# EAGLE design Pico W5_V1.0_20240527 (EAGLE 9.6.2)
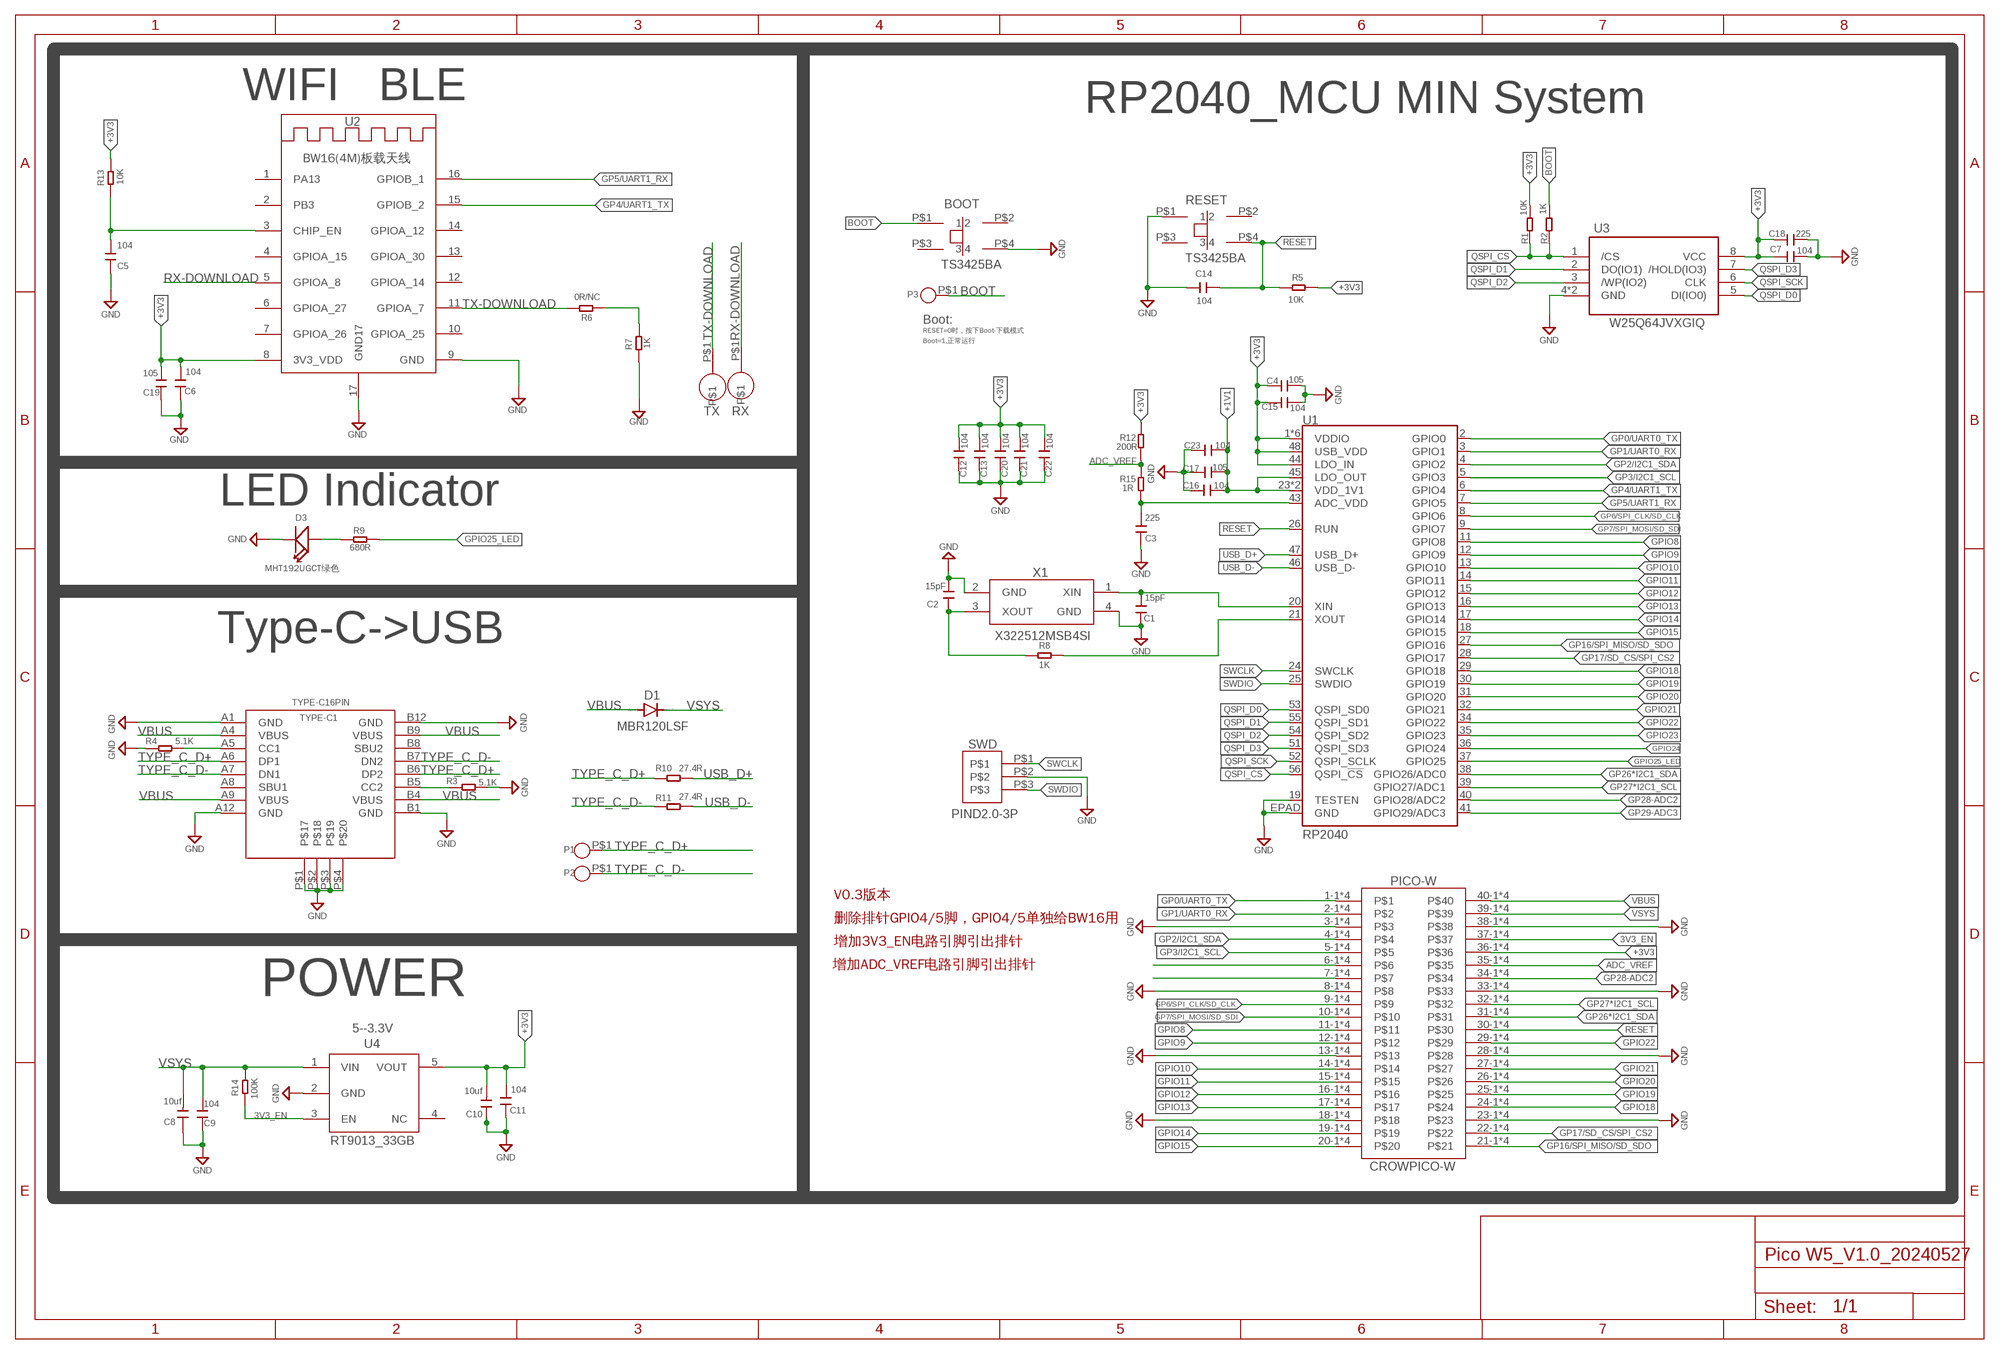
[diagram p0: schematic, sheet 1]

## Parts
BOOT  TS3425BA  KEY  [SMD_KEY4.2*3.*.2.5]
C1  15pF  C0201  [0201_W]
C2  15pF  C0201  [0201_W]
C3  225  C0201  [0201_W]
C4  105  C0201  [0201_W]
C5  104  C0201  [0201_W]
C6  104  C0201  [0201_W]
C7  104  C0201  [0201_W]
C8  10uf  C0402  [0402]
C9  104  C0402  [0201_W]
C10  10uf  C0402  [0402]
C11  104  C0402  [0201_W]
C12  104  C0201  [0201_W]
C13  104  C0201  [0201_W]
C14  104  C0402  [0201_W]
C15  104  C0201  [0201_W]
C16  104  C0201  [0201_W]
C17  105  C0201  [0201_W]
C18  225  C0201  [0201_W]
C19  105  C0201  [0201_W]
C20  104  C0201  [0201_W]
C21  104  C0201  [0201_W]
C22  104  C0201  [0201_W]
C23  104  C0201  [0201_W]
D1  MBR120LSF  DIODE-SOD123  [SOD123]
D3  MHT192UGCT绿色  DISCRETE_007-LED0603  [DISCRETE_D0603]
P1  TP  CROWPICO_W_PAD-1P  [CROWPICO_W_PAD-1P]
P2  TP  CROWPICO_W_PAD-1P  [CROWPICO_W_PAD-1P]
P3  TP  CROWPICO_W_PAD-1P  [CROWPICO_W_PAD-1P]
PICO-W  CROWPICO-W  CROWPICO-WCROWPICO-W1  [CROWPICO-W]
R1  10K  R0201  [0201_W]
R2  1K  R0201  [0201_W]
R3  5.1K  R0201  [0201_W]
R4  5.1K  R0201  [0201_W]
R5  10K  R0201  [0201_W]
R6  0R/NC  R0201  [0201_W]
R7  1K  R0201  [0201_W]
R8  1K  R0201  [0201_W]
R9  680R  R0201  [0201_W]
R10  27.4R  R0201  [0201_W]
R11  27.4R  R0201  [0201_W]
R12  200R  R0201  [0201_W]
R13  10K  R0201  [0201_W]
R14  100K  R0201  [0201_W]
R15  1R  R0201  [0201_W]
RESET  TS3425BA  KEY  [SMD_KEY4.2*3.*.2.5]
RX  TP  [TP2]
SWD  PIND2.0-3P  PIND2.0  [HDR2.0-3P]
TX  TP  [TP2]
TYPE-C1  TYPE-C16PIN  TYPE-C-16PIN  [TYPE-C16PIN2MD(073)]
U1  RP2040  RP2040_RP2040  [RP2040_QFN-56]
U2  BW16(4M)板载天线  BW16  [BW16]
U3  W25Q64JVXGIQ  W25QXX  [W25QXX-XSON-8-EP(4X4)]
U4  RT9013_33GB  RT9013  [SOT23-5_W]
X1  X322512MSB4SI  A_XBJ_XTAL  [A_XBJ_SMD3225]

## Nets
3V3_EN: PICO-W.37-1 PICO-W.37-2 PICO-W.37-3 PICO-W.37-4 R14.1 U4.3(EN)
+1V1: C16.1 C17.1 C23.1 U1.23(VDD_1V1) U1.45(LDO_OUT) U1.50(VDD_1V1)
+3V3: C4.2 C6.2 C7.1 C10.2 C11.2 C12.1 C13.1 C15.2 C18.1 C19.2 C20.1 C21.1 C22.1 PICO-W.36-1 PICO-W.36-2 PICO-W.36-3 PICO-W.36-4 R1.2 R5.2 R12.2 R13.2 U1.1(VDDIO) U1.10(VDDIO) U1.22(VDDIO) U1.33(VDDIO) U1.42(VDDIO) U1.44(LDO_IN) U1.48(USB_VDD) U1.49(VDDIO) U2.8(3V3_VDD) U3.8(VCC) U4.5(VOUT)
ADC_VREF: PICO-W.35-1 PICO-W.35-2 PICO-W.35-3 PICO-W.35-4 R12.1 R15.2
BOOT: BOOT.P$1 P3.P$1 R2.2
GND: BOOT.P$4 C1.2 C2.1 C3.2 C4.1 C5.1 C6.1 C7.2 C8.1 C9.1 C10.1 C11.1 C12.2 C13.2 C14.1 C15.1 C16.2 C17.2 C18.2 C19.1 C20.2 C21.2 C22.2 C23.2 D3.- PICO-W.3-1 PICO-W.3-2 PICO-W.3-3 PICO-W.3-4 PICO-W.8-1 PICO-W.8-2 PICO-W.8-3 PICO-W.8-4 PICO-W.13-1 PICO-W.13-2 PICO-W.13-3 PICO-W.13-4 PICO-W.18-1 PICO-W.18-2 PICO-W.18-3 PICO-W.18-4 PICO-W.23-1 PICO-W.23-2 PICO-W.23-3 PICO-W.23-4 PICO-W.28-1 PICO-W.28-2 PICO-W.28-3 PICO-W.28-4 PICO-W.33-1 PICO-W.33-2 PICO-W.33-3 PICO-W.33-4 PICO-W.38-1 PICO-W.38-2 PICO-W.38-3 PICO-W.38-4 R3.2 R4.1 R7.1 RESET.P$1 SWD.P$2 TYPE-C1.A1(GND) TYPE-C1.A12(GND) TYPE-C1.B1(GND) TYPE-C1.B12(GND) TYPE-C1.P$1 TYPE-C1.P$2 TYPE-C1.P$3 TYPE-C1.P$4 U1.19(TESTEN) U1.EPAD(GND) U2.9(GND) U2.17(GND17) U3.4(GND) U3.EP(GND) U4.2(GND) X1.2(GND) X1.4(GND)
GP0/UART0_TX: PICO-W.1-1 PICO-W.1-2 PICO-W.1-3 PICO-W.1-4 U1.2(GPIO0)
GP1/UART0_RX: PICO-W.2-1 PICO-W.2-2 PICO-W.2-3 PICO-W.2-4 U1.3(GPIO1)
GP2/I2C1_SDA: PICO-W.4-1 PICO-W.4-2 PICO-W.4-3 PICO-W.4-4 U1.4(GPIO2)
GP3/I2C1_SCL: PICO-W.5-1 PICO-W.5-2 PICO-W.5-3 PICO-W.5-4 U1.5(GPIO3)
GP4/UART1_TX: U1.6(GPIO4) U2.15(GPIOB_2)
GP5/UART1_RX: U1.7(GPIO5) U2.16(GPIOB_1)
GP6/SPI_CLK/SD_CLK: PICO-W.9-1 PICO-W.9-2 PICO-W.9-3 PICO-W.9-4 U1.8(GPIO6)
GP7/SPI_MOSI/SD_SDI: PICO-W.10-1 PICO-W.10-2 PICO-W.10-3 PICO-W.10-4 U1.9(GPIO7)
GP16/SPI_MISO/SD_SDO: PICO-W.21-1 PICO-W.21-2 PICO-W.21-3 PICO-W.21-4 U1.27(GPIO16)
GP17/SD_CS/SPI_CS2: PICO-W.22-1 PICO-W.22-2 PICO-W.22-3 PICO-W.22-4 U1.28(GPIO17)
GP26*I2C1_SDA: PICO-W.31-1 PICO-W.31-2 PICO-W.31-3 PICO-W.31-4 U1.38(GPIO26/ADC0)
GP27*I2C1_SCL: PICO-W.32-1 PICO-W.32-2 PICO-W.32-3 PICO-W.32-4 U1.39(GPIO27/ADC1)
GP28-ADC2: PICO-W.34-1 PICO-W.34-2 PICO-W.34-3 PICO-W.34-4 U1.40(GPIO28/ADC2)
GP29-ADC3: U1.41(GPIO29/ADC3)
GPIO8: PICO-W.11-1 PICO-W.11-2 PICO-W.11-3 PICO-W.11-4 U1.11(GPIO8)
GPIO9: PICO-W.12-1 PICO-W.12-2 PICO-W.12-3 PICO-W.12-4 U1.12(GPIO9)
GPIO10: PICO-W.14-1 PICO-W.14-2 PICO-W.14-3 PICO-W.14-4 U1.13(GPIO10)
GPIO11: PICO-W.15-1 PICO-W.15-2 PICO-W.15-3 PICO-W.15-4 U1.14(GPIO11)
GPIO12: PICO-W.16-1 PICO-W.16-2 PICO-W.16-3 PICO-W.16-4 U1.15(GPIO12)
GPIO13: PICO-W.17-1 PICO-W.17-2 PICO-W.17-3 PICO-W.17-4 U1.16(GPIO13)
GPIO14: PICO-W.19-1 PICO-W.19-2 PICO-W.19-3 PICO-W.19-4 U1.17(GPIO14)
GPIO15: PICO-W.20-1 PICO-W.20-2 PICO-W.20-3 PICO-W.20-4 U1.18(GPIO15)
GPIO18: PICO-W.24-1 PICO-W.24-2 PICO-W.24-3 PICO-W.24-4 U1.29(GPIO18)
GPIO19: PICO-W.25-1 PICO-W.25-2 PICO-W.25-3 PICO-W.25-4 U1.30(GPIO19)
GPIO20: PICO-W.26-1 PICO-W.26-2 PICO-W.26-3 PICO-W.26-4 U1.31(GPIO20)
GPIO21: PICO-W.27-1 PICO-W.27-2 PICO-W.27-3 PICO-W.27-4 U1.32(GPIO21)
GPIO22: PICO-W.29-1 PICO-W.29-2 PICO-W.29-3 PICO-W.29-4 U1.34(GPIO22)
GPIO23: U1.35(GPIO23)
GPIO24: U1.36(GPIO24)
GPIO25_LED: R9.2 U1.37(GPIO25)
N$1: C2.2 R8.1 X1.3(XOUT)
N$2: R8.2 U1.21(XOUT)
N$3: C1.1 U1.20(XIN) X1.1(XIN)
N$4: C3.1 R15.1 U1.43(ADC_VDD)
N$5: R3.1 TYPE-C1.B5(CC2)
N$7: R6.1 R7.2
N$8: PICO-W.6-1 PICO-W.6-2 PICO-W.6-3 PICO-W.6-4
N$9: PICO-W.7-1 PICO-W.7-2 PICO-W.7-3 PICO-W.7-4
N$14: R4.2 TYPE-C1.A5(CC1)
N$16: C5.2 R13.1 U2.3(CHIP_EN)
N$35: D3.+ R9.1
QSPI_CS: R1.1 R2.1 U1.56(QSPI_!CS!) U3.1(/CS)
QSPI_D0: U1.53(QSPI_SD0) U3.5(DI(IO0))
QSPI_D1: U1.55(QSPI_SD1) U3.2(DO(IO1))
QSPI_D2: U1.54(QSPI_SD2) U3.3(/WP(IO2))
QSPI_D3: U1.51(QSPI_SD3) U3.7(/HOLD(IO3))
QSPI_SCK: U1.52(QSPI_SCLK) U3.6(CLK)
RESET: C14.2 PICO-W.30-1 PICO-W.30-2 PICO-W.30-3 PICO-W.30-4 R5.1 RESET.P$4 U1.26(RUN)
RX-DOWNLOAD: RX.P$1 U2.5(GPIOA_8)
SWCLK: SWD.P$1 U1.24(SWCLK)
SWDIO: SWD.P$3 U1.25(SWDIO)
TX-DOWNLOAD: R6.2 TX.P$1 U2.11(GPIOA_7)
TYPE_C_D+: P1.P$1 R10.1 TYPE-C1.A6(DP1) TYPE-C1.B6(DP2)
TYPE_C_D-: P2.P$1 R11.1 TYPE-C1.A7(DN1) TYPE-C1.B7(DN2)
USB_D+ [USB]: R10.2 U1.47(USB_D+)
USB_D- [USB]: R11.2 U1.46(USB_D-)
VBUS [PWR]: D1.A PICO-W.40-1 PICO-W.40-2 PICO-W.40-3 PICO-W.40-4 TYPE-C1.A4(VBUS) TYPE-C1.A9(VBUS) TYPE-C1.B4(VBUS) TYPE-C1.B9(VBUS)
VSYS: C8.2 C9.2 D1.C PICO-W.39-1 PICO-W.39-2 PICO-W.39-3 PICO-W.39-4 R14.2 U4.1(VIN)
Unconnected: BOOT.P$2 BOOT.P$3 RESET.P$2 RESET.P$3 TYPE-C1.A8(SBU1) TYPE-C1.B8(SBU2) U2.1(PA13) U2.2(PB3) U2.4(GPIOA_15) U2.6(GPIOA_27) U2.7(GPIOA_26) U2.10(GPIOA_25) U2.12(GPIOA_14) U2.13(GPIOA_30) U2.14(GPIOA_12) U4.4(NC)

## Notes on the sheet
- WIFI   BLE | RP2040_MCU MIN System
- Boot:
- RESET=0时，按下Boot-下载模式
- Boot=1,正常运行
- LED Indicator
- Type-C->USB
- V0.3版本
- 删除排针GPIO4/5脚，GPIO4/5单独给BW16用
- 增加3V3_EN电路引脚引出排针
- 增加ADC_VREF电路引脚引出排针
- POWER
- 5--3.3V

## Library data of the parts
BOOT RESET = CKP:KEY
C1-C7 C12 C13 C15-C23 = WGH:C0201
C8 C10 = A_xbj:C0402
C9 C11 C14 = WGH:C0402
D1 = diode:DIODE-: DIODE
D3 = Crowtail_SIM1606:DISCRETE_007-LED*
P1-P3 = ESP32- 3.5 TFT Display(RGB)-V2.0:CROWPICO_W_PAD-1P
PICO-W = CKP:CROWPICO-W
R1-R15 = WGH:R0201
RX TX = CKP:TP
SWD = CKP:PIND2.0
TYPE-C1 = CKP:TYPE-C-16PIN
U1 = Lora_RA-08H_Dev:RP2040_RP2040: Raspberry Pi RP2040 MCU 56-pin 32-bit Microcontroller with 264kB of SRAM and external flash support up to 16MB Getting Started with the RP2040 Dual-core ARM Cortex M0+ processor, flexible clock running up to 133 MHz 264kB of SRAM, and QSPI control of common flash memory USB 1.1 Host and Device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; PROD_ID: IC-15502
U2 = CKP:BW16
U3 = CKP:W25QXX
U4 = WGH:RT9013
X1 = CrowBot_V1.4:A_XBJ_XTAL

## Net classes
0 default: width 0.102 mm, drill 0.254 mm, clearance 0.102 mm
1 PWR: width 0.254 mm
2 GND: width 0.203 mm
3 RS485: width 0.203 mm, clearance 0.203 mm
4 USB: width 0.152 mm, clearance 0.152 mm
5 ANT: width 0.889 mm, clearance 0.203 mm
6 DVI-D0: width 0.203 mm, clearance 0.203 mm to class 0, clearance 0.203 mm

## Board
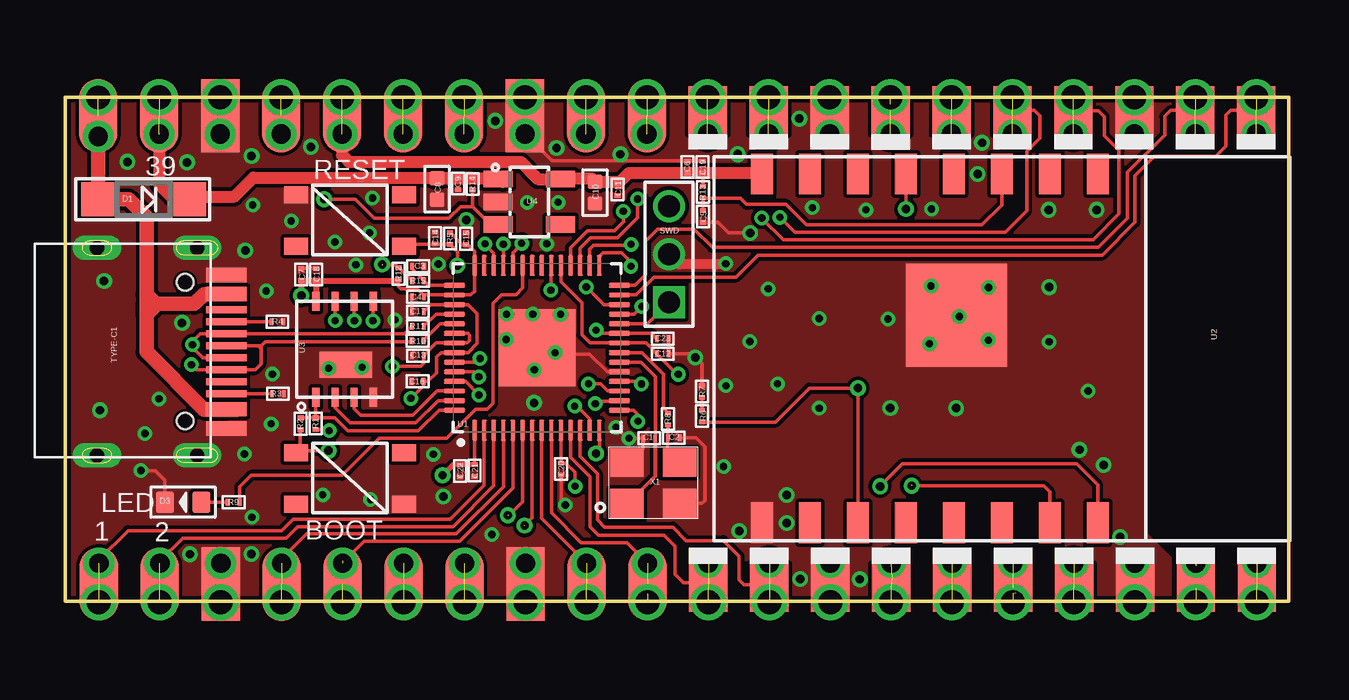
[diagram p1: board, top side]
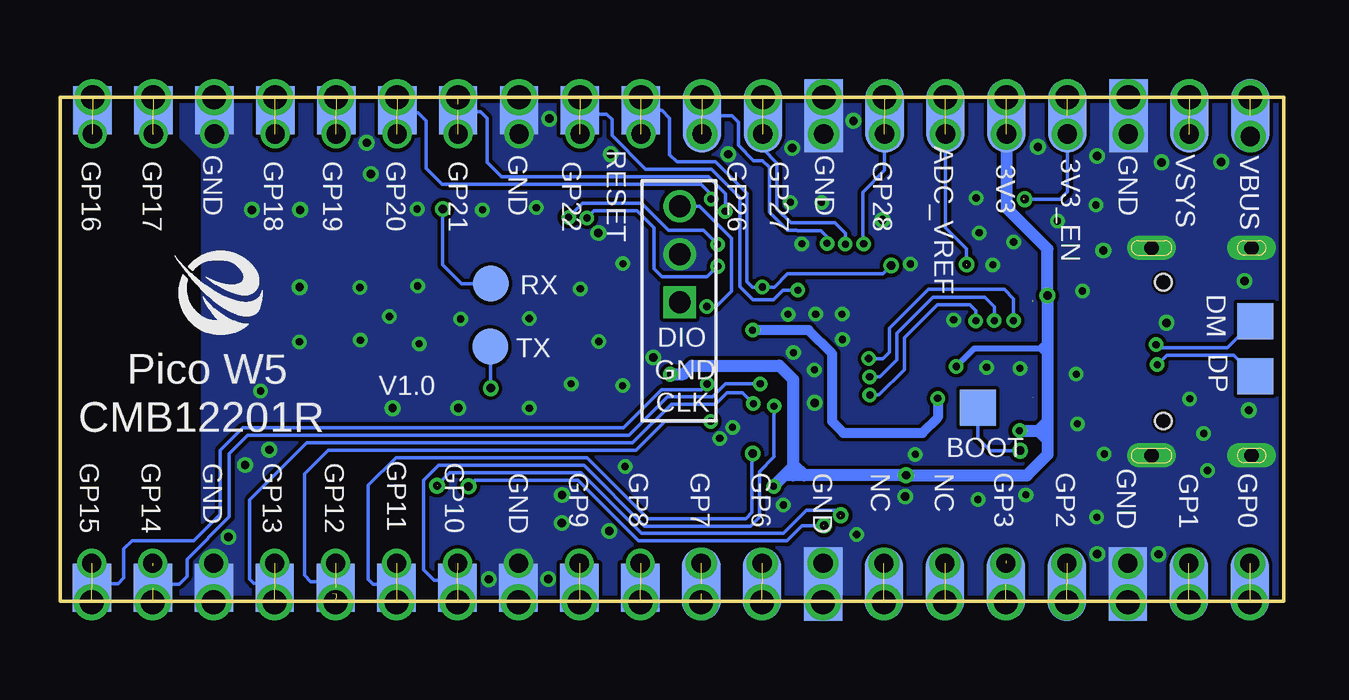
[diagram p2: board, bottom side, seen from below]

Size 51 x 21 mm. Coordinates in mm from the lower left corner, seen from the top.
Copper layers (1*16): Top 0.035mm / dielectric 1.5mm / Bottom 0.035mm
Design rules "default1 *": minimum track width 6mil, minimum drill 0.3mm, track to track 6mil, track to pad 4mil, pad to pad 4mil, via to via 6mil, smd to smd 6mil, copper to edge 6mil, drill to drill 4mil, minimum pad ring 6mil, minimum via ring 6mil, stop-mask expansion 4mil, vias tented up to drill 100mil, thermal gap 10mil
tRestrict: 6 lines
bRestrict: 6 lines

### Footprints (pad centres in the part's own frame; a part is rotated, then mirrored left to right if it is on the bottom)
SMD_KEY4.2*3.*.2.5 = smd 1 x 0.7: P$1 -2.184,0.102; P$2 2.316,0.102; P$3 -2.184,-2.048; P$4 2.316,-2.048
0201_W = smd 0.2 x 0.3: 1 -0.25,0; 2 0.25,0
0402 = smd 0.6 x 0.6: 1 -0.45,0; 2 0.45,0
SOD123 = smd 1.4 x 1.4: A 1.9,0; C -1.9,0
DISCRETE_D0603 = smd 0.762 x 0.889: + -0.762,0; - 0.762,0
CROWPICO_W_PAD-1P = smd 1.5 x 1.5: P$1 0,0
CROWPICO-W = smd 3.048 x 1.6: 1-1 -10.185,26.289; 2-1 -10.185,23.749; 3-1 -10.185,21.209; 4-1 -10.195,18.669; 5-1 -10.185,16.129; 6-1 -10.185,13.589; 7-1 -10.185,11.049; 8-1 -10.185,8.509; 9-1 -10.185,5.969; 10-1 -10.185,3.429; 31-1 9.322,3.454; 32-1 9.322,5.994; 33-1 9.322,8.534; 34-1 9.322,11.074; 35-1 9.322,13.614; 36-1 9.322,16.154; 37-1 9.322,18.694; 38-1 9.322,21.234; 39-1 9.322,23.774; 40-1 9.322,26.314 | smd 3.048 x 1.6 bottom: 1-2 -10.185,26.289; 2-2 -10.185,23.749; 3-2 -10.185,21.209; 4-2 -10.195,18.669; 5-2 -10.185,16.129; 6-2 -10.185,13.589; 7-2 -10.185,11.049; 8-2 -10.185,8.509; 9-2 -10.185,5.969; 10-2 -10.185,3.429; 31-2 9.322,3.454; 32-2 9.322,5.994; 33-2 9.322,8.534; 34-2 9.322,11.074; 35-2 9.322,13.614; 36-2 9.322,16.154; 37-2 9.322,18.694; 38-2 9.322,21.234; 39-2 9.322,23.774; 40-2 9.322,26.314 | drill 0.8 pad 1.295: 1-3 -9.322,26.289; 2-3 -9.322,23.749; 3-3 -9.322,21.209; 4-3 -9.322,18.669; 5-3 -9.322,16.129; 6-3 -9.322,13.589; 7-3 -9.322,11.049; 8-3 -9.322,8.509; 9-3 -9.322,5.969; 10-3 -9.322,3.429; 31-3 8.56,3.454; 32-3 8.56,5.994; 33-3 8.56,8.534; 34-3 8.56,11.074; 35-3 8.56,13.614; 36-3 8.56,16.154; 37-3 8.56,18.694; 38-3 8.56,21.234; 39-3 8.56,23.774; 40-3 8.458,26.314 | drill 1 pad 1.295: 1-4 -10.947,26.289; 2-4 -10.947,23.749; 3-4 -10.947,21.209; 4-4 -10.947,18.669; 5-4 -10.947,16.129; 6-4 -10.947,13.589; 7-4 -10.947,11.049; 8-4 -10.947,8.509; 9-4 -10.947,5.969; 10-4 -10.947,3.429; 11-4 -10.947,0.889; 12-4 -10.947,-1.651; 13-4 -10.947,-4.191; 14-4 -10.947,-6.731; 15-4 -10.947,-9.271; 16-4 -10.947,-11.811; 17-4 -10.947,-14.351; 18-4 -10.947,-16.891; 19-4 -10.947,-19.431; 20-4 -10.947,-21.971; 21-4 10.084,-21.946; 22-4 10.084,-19.406; 23-4 10.084,-16.866; 24-4 10.084,-14.326; 25-4 10.084,-11.786; 26-4 10.084,-9.246; 27-4 10.084,-6.706; 28-4 10.084,-4.166; 29-4 10.084,-1.626; 31-4 10.084,3.454; 32-4 10.084,5.994; 33-4 10.084,8.534; 34-4 10.084,11.074; 35-4 10.084,13.614; 36-4 10.084,16.154; 37-4 10.084,18.694; 38-4 10.084,21.234; 39-4 10.084,23.774 | smd 2.007 x 1.6: 11-1 -10.338,0.889; 12-1 -10.338,-1.651; 13-1 -10.338,-4.191; 14-1 -10.338,-6.731; 15-1 -10.338,-9.271; 16-1 -10.338,-11.811; 17-1 -10.338,-14.351; 18-1 -10.338,-16.891; 19-1 -10.338,-19.431; 20-1 -10.338,-21.971; 21-1 9.55,-21.946; 22-1 9.55,-19.406; 23-1 9.55,-16.866; 24-1 9.55,-14.326; 25-1 9.55,-11.786; 26-1 9.55,-9.246; 27-1 9.55,-6.706; 28-1 9.55,-4.166; 29-1 9.55,-1.626; 30-1 9.55,0.914 | smd 2.007 x 1.6 bottom: 11-2 -10.338,0.889; 12-2 -10.338,-1.651; 13-2 -10.338,-4.191; 14-2 -10.338,-6.731; 15-2 -10.338,-9.271; 16-2 -10.338,-11.811; 17-2 -10.338,-14.351; 18-2 -10.338,-16.891; 19-2 -10.338,-19.431; 20-2 -10.338,-21.971; 21-2 9.55,-21.946; 22-2 9.55,-19.406; 23-2 9.55,-16.866; 24-2 9.55,-14.326; 25-2 9.55,-11.786; 26-2 9.55,-9.246; 27-2 9.55,-6.706; 28-2 9.55,-4.166; 29-2 9.55,-1.626; 30-2 9.55,0.914 | drill 0.8 pad 0.813: 11-3 -9.322,0.889; 12-3 -9.322,-1.651; 13-3 -9.322,-4.191; 14-3 -9.322,-6.731; 15-3 -9.322,-9.271; 16-3 -9.322,-11.811; 17-3 -9.322,-14.351; 18-3 -9.322,-16.891; 19-3 -9.322,-19.431; 20-3 -9.322,-21.971; 21-3 8.56,-21.946; 22-3 8.56,-19.406; 23-3 8.56,-16.866; 24-3 8.56,-14.326; 25-3 8.56,-11.786; 26-3 8.56,-9.246; 27-3 8.56,-6.706; 28-3 8.56,-4.166; 29-3 8.56,-1.626; 30-3 8.56,0.914 | drill 1 pad 1.499: 30-4 10.084,0.914 | drill 0.991 pad 1.295: 40-4 10.084,26.314
TP2 = smd 1.5 x 1.5: P$1 0,0
HDR2.0-3P = drill 0.9 square: P$1 0,0 | drill 0.9: P$2 2,0; P$3 4,0
TYPE-C16PIN2MD(073) = smd 0.3 x 1.7: A1 -3.35,4.31; A4 -2.55,4.31; A5 -1.25,4.31; A6 -0.25,4.31; A7 0.25,4.31; A8 1.25,4.31; A9 2.55,4.31; A12 3.35,4.31; B1 3.05,4.31; B4 2.25,4.31; B5 1.75,4.31; B6 0.75,4.31; B7 -0.75,4.31; B8 -1.75,4.31; B9 -2.25,4.31; B12 -3.05,4.31 | drill 0.6 pad 1.016 long: P$1 -4.325,3.09; P$2 4.325,3.09; P$3 -4.325,-1.09; P$4 4.325,-1.09 | hole 0.68: -2.89,2.59; 2.89,2.59
RP2040_QFN-56 = smd 0.875 x 0.2: 1 -3.437,2.6; 2 -3.437,2.2; 3 -3.437,1.8; 4 -3.437,1.4; 5 -3.437,1; 6 -3.437,0.6; 7 -3.437,0.2; 8 -3.437,-0.2; 9 -3.437,-0.6; 10 -3.437,-1; 11 -3.437,-1.4; 12 -3.437,-1.8; 13 -3.437,-2.2; 14 -3.437,-2.6; 29 3.437,-2.6; 30 3.437,-2.2; 31 3.437,-1.8; 32 3.437,-1.4; 33 3.437,-1; 34 3.437,-0.6; 35 3.437,-0.2; 36 3.437,0.2; 37 3.437,0.6; 38 3.437,1; 39 3.437,1.4; 40 3.437,1.8; 41 3.437,2.2; 42 3.437,2.6 | smd 0.2 x 0.875: 15 -2.6,-3.437; 16 -2.2,-3.437; 17 -1.8,-3.437; 18 -1.4,-3.437; 19 -1,-3.437; 20 -0.6,-3.437; 21 -0.2,-3.437; 22 0.2,-3.437; 23 0.6,-3.437; 24 1,-3.437; 25 1.4,-3.437; 26 1.8,-3.437; 27 2.2,-3.437; 28 2.6,-3.437; 43 2.6,3.437; 44 2.2,3.437; 45 1.8,3.437; 46 1.4,3.437; 47 1,3.437; 48 0.6,3.437; 49 0.2,3.437; 50 -0.2,3.437; 51 -0.6,3.437; 52 -1,3.437; 53 -1.4,3.437; 54 -1.8,3.437; 55 -2.2,3.437; 56 -2.6,3.437 | smd 3.2 x 3.2: EPAD 0,0
BW16 = smd 1.7 x 0.9: 1 -6.9,5.84; 2 -6.9,3.84; 3 -6.9,1.84; 4 -6.9,-0.16; 5 -6.9,-2.16; 6 -6.9,-4.16; 7 -6.9,-6.16; 8 -6.9,-8.16; 9 7.626,-8.16; 10 7.626,-6.16; 11 7.626,-4.16; 12 7.626,-2.16; 13 7.626,-0.16; 14 7.626,1.84; 15 7.626,3.84; 16 7.626,5.84 | smd 4.3 x 4.2: 17 -1.02,-0.06
W25QXX-XSON-8-EP(4X4) = smd 0.8 x 0.3: 1 -2,1.2; 2 -2,0.4; 3 -2,-0.4; 4 -2,-1.2; 5 2,-1.2; 6 2,-0.4; 7 2,0.4; 8 2,1.2 | smd 1.067 x 2.184: EP -0.646,-0.051
SOT23-5_W = smd 0.69 x 1.2: 1 -0.95,-1.3; 2 0,-1.3; 3 0.95,-1.3; 4 0.95,1.3; 5 -0.95,1.3
A_XBJ_SMD3225 = smd 1.4 x 1.2: 1 -1.1,-0.85; 2 1.1,-0.85; 3 1.1,0.85; 4 -1.1,0.85

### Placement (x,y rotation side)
BOOT  11.81,6.08 0 top
C1  24.34,6.79 180 top
C2  25.36,6.8 180 top
C3  14.71,13.96 0 top
C4  14.7,12.68 0 top
C5  26.59,16.03 90 top
C6  25.95,18.09 270 top
C7  9.84,13.61 90 top
C8  15.5,17.17 90 top
C9  16.38,17.39 90 top
C10  22.08,17.02 90 top
C11  23.03,17.16 90 top
C12  24.9,10.3 0 top
C13  14.69,10.23 180 top
C14  15.43,15.12 270 top
C15  16.71,15.1 270 top
C16  14.69,9.15 180 top
C17  14.69,12.06 180 top
C18  10.46,13.61 90 top
C19  26.58,18.09 270 top
C20  20.66,5.5 270 top
C21  17.07,5.43 270 top
C22  16.45,5.43 270 top
C23  24.91,10.93 0 top
D1  3.28,16.74 180 top
D3  4.92,4.12 180 top
P1  1.19,9.36 270 bottom
P2  1.19,11.67 270 bottom
P3  12.74,8.06 270 bottom
PICO-W  27.7,10.9 90 top
R1  10.44,7.4 270 top
R2  9.81,7.39 270 top
R3  8.87,8.63 0 top
R4  8.85,11.64 180 top
R5  16.04,15.11 90 top
R6  26.56,7.71 270 top
R7  26.55,8.73 270 top
R8  25.13,7.59 90 top
R9  7.03,4.12 0 top
R10  14.69,10.84 0 top
R11  14.7,11.45 0 top
R12  13.89,13.64 270 top
R13  26.59,17.04 90 top
R14  16.99,17.38 90 top
R15  14.71,13.35 180 top
RESET  11.81,16.83 0 top
RX  33.05,13.23 0 bottom
SWD  25.17,12.45 90 top
TX  33.07,10.6 0 bottom
TYPE-C1  2.42,10.39 270 top
U1  19.67,10.55 90 top
U2  37.21,10.89 270 top
U3  11.65,10.49 90 top
U4  19.35,16.64 270 top
X1  24.51,4.92 0 top

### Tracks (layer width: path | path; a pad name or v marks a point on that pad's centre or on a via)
3V3_EN  (via drill 0.35)  (3 unrouted)
  Top 0.152: R14.1 16.99,16.43 | 16.99,16.43 17.73,15.69 U4.3 | PICO-W.37-2 PICO-W.37-3 | v10.8,16.75 12.09,16.75 12.89,15.94 15.99,15.94 16.48,16.43 16.99,16.43
  Bottom 0.152: PICO-W.37-2 9.01,17.05 9.32,16.74 10.86,16.74
+1V1  (via drill 0.3 pad 0.6)
  Top 0.152: C17.1 15.24,12.35 U1.45 16.79,12.35 17.18,11.97 17.18,10.74 16.79,10.35 U1.50 15.66,10.35 15.48,10.17 15.48,9.51 15.12,9.15 C16.1 14.94,8.97 v14.42,8.45 v14.41,8.45 | C23.1 24.44,11.15 U1.23 22.27,11.15 v22.13,11.29
  Bottom 0.406: v14.41,8.45 14.41,7.64 15.04,7.01 18.35,7.01 18.81,7.47 18.81,10.3 19.79,11.29 v22.13,11.29
+3V3  (via drill 0.3 pad 0.6, 0.35)  (4 unrouted)
  Top 0.152: U1.1 C21.1 | U1.10 C20.1 | 15.02,12.75 U1.44 16.9,12.75 17.07,12.92 U1.42 17.07,14.58 16.79,14.85 C15.2 16.55,14.85 R5.2 | 15.02,12.75 14.93,12.75 14.67,13.01 13.98,13.01 13.9,13.09 R12.2 13.85,13.35 | U1.48 16.79,11.15 16.87,11.08 16.87,10.86 16.76,10.75 U1.49 15.47,10.75 C13.1 14.95,9.91 14.81,9.78 v13.64,9.78 | R1.2 10.97,7.15 v11.01,7.1 | 20.67,5.74 C20.1 20.87,5.75 21.26,5.36 v21.26,4.78 | U1.33 20.67,13.31 21.55,12.43 21.55,11.09 21.88,10.75 U1.22 24.2,10.75 C12.1 25.51,9.45 v25.56,9.45 | 26.59,17.83 C19.2 | R13.2 26.59,17.83 | 26.68,17.84 26.67,17.83 26.59,17.83 | 9.88,13.35 9.84,13.35 C7.1 | 27.24,17.84 29,17.84 U2.8 | 10.27,13.35 C18.1 10.47,13.35 13.09,13.35 13.08,13.36 | 15.02,12.75 C4.2
  Top 0.2: C21.1 16.46,5.68 C22.1 16.17,5.68 v15.74,5.24 | C20.1
  Top 0.254: 10.46,12.5 C18.1 | 26.59,17.75 26.68,17.84 | C18.1 10.27,13.35 9.88,13.35 9.84,13.32 v9.84,12.73 | C18.1 13.86,13.35 R12.2
  Top 0.508: 29.05,17.86 29.03,17.84 27.24,17.84 26.68,17.84 C6.2 23.51,17.84 23.07,17.41 | PICO-W.36-1 11.55,18.59 11.84,18.3 18.99,18.3 19.7,17.59 U4.5 | 20.75,17.49 U4.5 | U4.5 20.67,17.6 21.95,17.6 C10.2 23.01,17.47 23.07,17.41 | C11.2 23.07,17.41
  Bottom 0.254: v13.64,9.78 12.89,10.53 10.15,10.53 | 10.15,10.53 9.84,10.53 | 10.15,10.53 | 10.15,10.53 9.84,10.83 | 10.15,10.53 9.84,10.22
  Bottom 0.508: PICO-W.36-1 11.55,16.38 9.84,14.68 v9.84,12.73 9.84,10.83 9.84,10.53 9.84,10.22 9.84,7.47 | 19.98,5.24 v15.74,5.24 10.7,5.24 9.84,6.1 9.84,6.72 | v25.56,9.45 25.01,9.45 24.65,9.81 21.02,9.81 20.45,9.24 20.45,5.71 | 20.45,5.59 20.45,5.24 | 20.45,5.71 19.98,5.24 | 20.45,5.71 20.45,5.59 | 20.45,5.59 20.8,5.24 | 20.8,5.24 v21.26,4.78 | 19.98,5.24 20.8,5.24 | 9.84,7.47 9.84,7.1 | 9.84,7.1 9.84,6.72 | v11.01,7.1 10.21,7.1 | 10.21,7.1 9.84,7.1 | 9.84,7.47 10.21,7.1 | 10.21,7.1 10.21,7.09 9.84,6.72
ADC_VREF  (via drill 0.35)  (5 unrouted)
  Top 0.152: R15.2 13.92,13.89 R12.1 13.79,13.99 13.22,13.99
  Bottom 0.152: 13.22,13.99 13.22,14.69 14.09,15.55 PICO-W.35-1
  other vias: 13.21,14.03
BOOT  (via drill 0.35)
  Top 0.152: R2.2 9.8,7.13 9.8,6.37 BOOT.P$1 9.71,6.27 v10.98,6.27
  Bottom 0.152: P3.P$1 12.74,6.78 12.23,6.27 v10.98,6.27
GND  (via drill 0.3, 0.3 pad 0.6, 0.35)
  Top 0.152: C23.2 C12.2 26.15,10.3 26.55,9.9 R7.1 | U1.19 22.6,9.55 21.87,10.29 20.95,10.29 | 20.95,10.29 20.39,10.29 | 20.31,10.19 20.4,10.19 20.03,10.55 U1.EPAD | C20.2 20.67,4.19 v20.85,4.01 | C2.1 26.29,6.8 26.67,6.42 26.67,4.18 26.56,4.07 X1.2 | C19.1 C6.1 20.29,18.34 PICO-W.33-3 | 27.12,14.03 27.54,14.03 | C5.1 27.22,15.78 27.66,15.34 v28.56,15.34 | PICO-W.28-1 PICO-W.28-3 | C17.2 C4.1 14.43,12.69 | C7.2 C18.2 | v22.96,7.24 23.41,6.79 C1.2 24.09,6.34 23.53,5.77 X1.4 | 19.02,11.62 19.02,11.2 U1.EPAD | 19.15,10.11 19.22,10.11 U1.EPAD | U1.EPAD 20.68,10.55 20.95,10.29 | U1.EPAD 20.71,9.51 20.75,9.51 | 9.1,8.65 R3.2 | v3.16,5.44 3.75,5.44 4.16,5.04 D3.-
  Top 0.406: SWD.P$2 25.19,14.45 25.61,14.03 27.12,14.03 27.51,14.03 v27.53,14.06
  other vias: 27.44,5.61 15.77,4.36 8.59,7.38 8.38,12.92 20.55,16.62 19.26,16.62 7.82,16.5 12.82,16.79 19.56,9.64 31.15,16.39 33.39,16.3 36.11,16.33 19.55,8.26 29.31,13.01 28.54,10.81 27.55,8.97 7.78,3.5 3.33,6.98 3.91,8.43 31.43,8.04 30.07,4.42 43.28,5.67 37.14,8.04 40.99,16.3 7.51,14.6 4.88,11.59 30.61,20.1 38.22,19.1 20.48,18.87 17.93,20.01 5.09,18.28 7.77,18.55 10.24,18.93 2.6,18.3 5.21,1.95 7.76,1.96 30.65,0.92 33.13,0.91 26.27,10.15 29.69,9.05 43,16.3 34.4,8.04 38.04,17.79 43.98,2.67 1.63,13.34 1.45,7.95 20.43,10.35 11.25,14.97 12.69,15.35 8.64,9.46 12.12,14.01 10.99,9.7 12.37,9.74 36.09,13.13 38.5,13.07 36.03,10.72 37.27,11.85 34.3,11.76 31.43,11.77 17.79,2.77 16.72,15.88 13.75,11.72 18.41,11.95 20.65,11.95 19.5,11.96 18.39,10.9 15.55,14.04 20.08,14.89 23.15,18.62 41.01,13.08 38.48,10.87 41.02,10.8 42.64,8.75 15.35,6.11 7.47,6.13 28.04,18.62 23.5,6.78 30.08,3.26 10.74,4.43 42.28,6.31 12.73,4.23 9.42,15.84 28.1,2.92
  pour Bottom (no thermals): 0.05,21.01 45.95,21.01 45.95,19.31 45.05,18.41 45.05,2.81 45.95,1.91 45.95,0.01 0.05,0.01
  pour Top (no thermals): 0.05,21.01 46.05,21.01 46.05,19.51 45.05,18.51 45.05,2.81 46.05,1.81 46.05,0.01 0.05,0.01
GP0/UART0_TX  (3 unrouted)
  Top 0.152: U1.2 17.47,4.83 16.05,3.41 9.7,3.41 | PICO-W.1-1 1.41,1.73 2.62,2.94 9.02,2.94 9.5,3.41 9.7,3.41 | 9.7,3.41
GP1/UART0_RX  (3 unrouted)
  Top 0.152: U1.3 17.87,4.8 16.17,3.11 9.7,3.11 9.21,2.62 4.9,2.62 3.95,1.67 PICO-W.2-2
GP2/I2C1_SDA  (3 unrouted)
  Top 0.152: U1.4 18.27,4.77 16.3,2.8 10.08,2.8 9.03,1.76 PICO-W.4-1
GP3/I2C1_SCL  (3 unrouted)
  Top 0.152: 11.57,1.69 PICO-W.5-2 11.57,1.61 12.46,2.5 16.43,2.5 18.67,4.73 U1.5
GP4/UART1_TX  (via drill 0.35)  (2 unrouted)
  Top 0.152: 18.48,3.56 19.07,4.15 U1.6 | v35.28,4.8 40.79,4.8 41.05,4.55 U2.15
  Bottom 0.152: v18.46,3.58 18.66,3.78 19.88,3.78 20.84,2.82 26.75,2.82 29.28,5.35 34.77,5.35 35.29,4.83
GP5/UART1_RX  (via drill 0.35)  (1 unrouted)
  Top 0.152: v19.16,3.15 19.47,3.46 U1.7 | U2.16 43.05,4.84 42.17,5.72 34.91,5.72 v33.97,4.78
  Bottom 0.152: v19.15,3.15 v19.15,3.14 20.06,3.14 20.7,2.51 26.88,2.51 29.41,5.04 33.28,5.04 33.6,5.04 33.72,5.04 v33.97,4.78
GP6/SPI_CLK/SD_CLK  (3 unrouted)
  Top 0.152: U1.8 19.87,3.44 PICO-W.9-3
GP7/SPI_MOSI/SD_SDI  (3 unrouted)
  Top 0.152: U1.9 20.27,3.67 21.51,2.43 23.43,2.43 PICO-W.10-3 | PICO-W.10-3 24.47,1.39 24.27,1.2 PICO-W.10-1 | PICO-W.10-1 24.27,0.3 | PICO-W.10-1 PICO-W.10-3
GP16/SPI_MISO/SD_SDO  (3 unrouted)
  Top 0.152: U1.27 23.79,12.75 24.54,13.5 27.97,13.5 28.89,14.42 43.23,14.42 44.6,15.78 44.6,17.73 45.4,18.53 47.96,18.53 48.39,18.96 48.39,20.25 48.59,20.45 PICO-W.21-2
GP17/SD_CS/SPI_CS2  (3 unrouted)
  Top 0.152: U1.28 23.75,13.15 24.19,13.59 24.19,15 24.69,15.5 26.21,15.5 26.98,14.74 43.06,14.74 44.28,15.96 44.28,17.86 45.84,19.42 45.84,20.2 46.09,20.45 PICO-W.22-1
GP26*I2C1_SDA  (via drill 0.3 pad 0.6)  (3 unrouted)
  Top 0.152: 18.65,13.97 U1.38 18.67,14.52 19.03,14.88 v19.03,14.91
  Bottom 0.152: 24.1,19.46 PICO-W.31-3 24.29,19.42 24.03,19.42 | v19.03,14.91 19.03,15.18 19.29,15.44 20.26,15.44 20.27,15.46 20.67,15.46 21.42,16.21 21.42,18.07 21.71,18.36 22.08,18.36 22.73,19 22.73,19.95 23,20.22 PICO-W.31-2
GP27*I2C1_SCL  (via drill 0.3 pad 0.6)  (3 unrouted)
  Top 0.152: v18.26,14.87 v18.27,14.87 U1.39
  Bottom 0.152: v18.26,14.87 v18.26,14.88 18.26,15.32 18.7,15.76 20.54,15.76 21.11,16.33 21.11,18.25 21.71,18.85 PICO-W.32-2
GP28-ADC2  (via drill 0.3 pad 0.6)  (3 unrouted)
  Top 0.152: v17.5,14.89 17.5,14.86 17.87,14.49 U1.40
  Bottom 0.152: PICO-W.34-1 16.63,17.94 17.53,17.04 17.53,14.92 v17.5,14.89
GPIO8  (3 unrouted)
  Top 0.152: U1.11 21.07,5.99 21.88,5.18 21.88,3.09 22.24,2.74 24.97,2.74 25.43,2.28 25.43,1.11 25.77,0.77 26.6,0.77 PICO-W.11-2
GPIO9  (3 unrouted)
  Top 0.152: U1.12 21.47,6.03 22.18,5.31 22.18,3.38 22.49,3.08 25.33,3.08 25.89,2.52 27.44,2.52 28.1,1.87 28.1,0.9 28.3,0.69 29.18,0.69 29.3,0.57 29.3,0.38 29.35,0.33 PICO-W.12-2
GPIO10  (via drill 0.3 pad 0.6)  (4 unrouted)
  Top 0.152: v21.24,8.12 21.35,8.12 21.87,7.6 U1.13
  Bottom 0.152: v21.23,8.11 v21.24,8.12 21.24,6.01 21.85,5.4 21.85,3.5 22.23,3.12 26.63,3.12 29.16,5.65 35.22,5.65 35.84,5.04 35.84,1.3 35.4,0.86 34.46,0.86 34.41,0.91 34.46,0.95
GPIO11  (via drill 0.35)  (3 unrouted)
  Top 0.152: 22.28,7.11 U1.14 22.27,6.29 v22.13,6.15
  Bottom 0.152: PICO-W.15-1 36.97,0.71 37.95,0.71 38.15,0.91 38.15,4.82 37,5.97 29.03,5.97 26.49,3.43 22.42,3.43 22.16,3.69 22.16,6.12 v22.13,6.15
GPIO12  (via drill 0.3 pad 0.6)  (4 unrouted)
  Top 0.152: U1.15 23.68,7.95 23.87,7.76 v23.87,7.49
  Bottom 0.152: v23.88,7.49 v23.87,7.49 25.78,7.49 26.99,6.28 39.83,6.28 40.81,5.3 40.81,1.07 40.55,0.81 39.73,0.81 39.51,0.6 PICO-W.16-1 39.63,0.45 39.63,0.33 | 39.5,0.3 39.45,0.3
GPIO13  (via drill 0.3 pad 0.6)  (4 unrouted)
  Top 0.152: U1.16 23.09,8.34 22.21,8.34 v22.1,8.23
  Bottom 0.152: 42.05,0.33 42.05,0.74 42.93,0.74 43.09,0.9 43.09,4.21 40.72,6.59 27.14,6.59 25.52,8.2 23.67,8.2 23.19,8.68 22.55,8.68 v22.1,8.23
GPIO14  (via drill 0.3 pad 0.6)  (3 unrouted)
  Top 0.152: 47.13,1.41 PICO-W.19-2 47.13,1.47 | U1.17 22.61,8.75 22.32,9.05 v21.82,9.05
  Bottom 0.152: v21.82,9.05 23.25,9.05 23.8,8.51 25.69,8.51 27.29,6.9 43.18,6.9 43.95,6.14 43.95,3.51 45.71,1.75 45.71,1.04 46.04,0.71 47.12,0.71 47.24,0.83 47.24,0.67 PICO-W.19-2
GPIO15  (via drill 0.3 pad 0.6)  (3 unrouted)
  Top 0.152: 23.11,9.16 U1.18 23.91,9.15 v24.02,9.04
  Bottom 0.152: PICO-W.20-2 49.67,0.74 49.65,0.72 48.58,0.72 48.34,0.97 48.34,2.17 47.99,2.51 45.42,2.51 44.32,3.62 44.32,6.28 43.38,7.22 27.51,7.22 25.92,8.81 24.25,8.81 v24.02,9.04
GPIO18  (via drill 0.3 pad 0.6)  (3 unrouted)
  Top 0.152: U1.29 22.27,14.36 22.42,14.51 23.19,14.51 23.59,14.11 v23.59,13.95 | 42.36,20.42 42.58,20.42 | 42.58,20.42 43.08,20.42 43.32,20.18 43.32,19.39 43.93,18.78 43.93,16.13 42.85,15.06 29.94,15.06 v29.04,15.96 | PICO-W.24-2 42.55,20.45 42.58,20.42
  Bottom 0.152: v23.59,13.95 24.03,13.51 25.92,13.51 26.24,13.84 26.24,15.55 26.95,16.26 28.74,16.26 v29.04,15.96
GPIO19  (via drill 0.3 pad 0.6)  (3 unrouted)
  Top 0.152: U1.30 21.87,14.67 22.02,14.82 23.55,14.82 v23.59,14.86 | v29.8,15.99 30.42,15.37 39.2,15.37 40.09,16.26 40.09,18.74 40.64,19.29 40.64,20.23 40.41,20.46 PICO-W.25-2
  Bottom 0.152: v23.59,14.86 24.18,15.45 25.64,15.45 26.76,16.57 29.22,16.57 v29.8,15.99
GPIO20  (via drill 0.3)  (3 unrouted)
  Top 0.152: U1.31 21.47,14.7 21.9,15.13 23.02,15.13 23.87,15.98 v23.87,16.75 v23.86,16.76
  Bottom 0.152: PICO-W.26-1 36.95,20.34 36.06,20.34 35.74,20.01 35.74,18.04 35.07,17.37 24.28,17.37 23.86,16.96 v23.86,16.76
GPIO21  (via drill 0.3)  (3 unrouted)
  Top 0.152: U1.32 21.07,14.73 21.78,15.44 22.9,15.44 23.27,15.81 v23.27,16.24
  Bottom 0.152: v23.27,16.24 23.27,16.98 23.96,17.68 32.59,17.68 33.21,18.29 33.21,20.12 33.47,20.38 34.41,20.38 PICO-W.27-1 34.41,20.7
GPIO22  (via drill 0.3 pad 0.6)  (3 unrouted)
  Top 0.152: U1.34 20.26,12.97 v20.24,12.95
  Bottom 0.152: PICO-W.29-1 29.33,20.29 28.21,20.29 28,20.08 28,19.4 26.59,17.99 23.84,17.99 22.66,16.82 22.66,13.1 22.11,12.55 21.27,12.55 20.86,12.95 v20.24,12.95
GPIO25_LED
  Top 0.152: U1.37 19.07,13.05 18.79,12.77 18.19,12.77 17.83,12.42 17.83,8.24 17.58,8 17.12,8 15.9,6.79 13.09,6.79 11.54,5.24 7.75,5.24 7.28,4.77 R9.2
N$1
  Top 0.152: R8.1 25.13,6.81 C2.2 25.11,6.24 25.59,5.77 X1.3
N$2
  Top 0.152: U1.21 24.04,10.35 24.94,9.46 24.94,8.03 R8.2
N$3
  Top 0.152: U1.20 24,9.95 24.61,9.35 24.61,5.21 24.59,5.2 | X1.1 23.47,4.07 24.59,5.2 | C1.1 24.59,5.2
N$4
  Top 0.152: U1.43 15.16,13.15 R15.1 14.46,13.85 C3.1
N$5
  Top 0.152: R3.1 TYPE-C1.B5
  Top 0.203: TYPE-C1.B5
N$7
  Top 0.152: R6.1 26.55,7.97 R7.2
N$8  (3 unrouted)
N$9  (3 unrouted)
N$14
  Top 0.152: TYPE-C1.A5 R4.2
N$16
  Top 0.152: C5.2 R13.1 28.14,16.79 28.4,16.53 30.06,16.53 30.91,15.68 38.22,15.68 39.05,16.5 U2.3
N$35
  Top 0.152: D3.+ R9.1
QSPI_CS  (1 unrouted)
  Top 0.152: R1.1 | R1.1 10.44,7.64 R2.1 | U1.56 15.58,7.95 14.72,7.09 11.78,7.09 11.22,7.65 R1.1 | R1.1 U3.1
QSPI_D0  (via drill 0.3 pad 0.6)
  Top 0.152: U1.53 16.69,9.15 v17.24,8.59 | v12.83,11.68 12.83,12.47 U3.5
  Bottom 0.152: v17.24,8.59 16.86,8.59 15.81,9.64 15.81,10.96 14.43,12.34 13.08,12.34 12.83,12.09 v12.83,11.68
QSPI_D1
  Top 0.152: U1.55 15.54,8.35 14.61,7.42 11.89,7.42 11.25,8.06 U3.2
QSPI_D2
  Top 0.152: U1.54 15.5,8.75 14.49,7.74 12.33,7.74 12.05,8.02 U3.3
QSPI_D3  (via drill 0.3 pad 0.6)
  Top 0.152: U1.51 17.15,9.95 v17.3,10.1 | U3.7 11.26,12.49 v11.26,11.68
  Bottom 0.152: v17.3,10.1 16.69,10.1 16.43,10.36 16.43,11.36 14.81,12.99 11.65,12.99 11.26,12.6 v11.26,11.68
QSPI_SCK  (via drill 0.3 pad 0.6)
  Top 0.152: U1.52 17.04,9.55 v17.25,9.35 | v12.05,11.69 U3.6
  Bottom 0.152: v17.25,9.35 16.82,9.35 16.11,10.05 16.11,11.16 14.62,12.66 12.45,12.66 12.05,12.26 v12.05,11.69
RESET  (via drill 0.3 pad 0.6, 0.35)  (3 unrouted)
  Top 0.152: 15.44,14.88 C14.2 15.44,14.86 R5.1 | U1.26 22.46,12.35 v21.72,13.09 | R5.1 16.35,14.55 v16.35,13.98 | RESET.P$4 14.2,14.86 R5.1
  Bottom 0.152: v21.72,13.09 | v21.72,13.09 22.14,13.09 22.36,13.31 22.36,16.99 23.67,18.3 25.28,18.3 25.59,18.6 25.59,20.13 25.91,20.45 PICO-W.30-1 | v21.72,13.09 | v21.72,13.09 21.23,13.09 20.68,13.64 16.7,13.64 v16.35,13.98
RX-DOWNLOAD  (via drill 0.35)
  Top 0.152: v35.05,16.33 U2.5
  Bottom 0.152: RX.P$1 34.27,13.23 35.05,14.01 v35.05,16.33
SWCLK
  Top 0.152: U1.24 24.28,11.55 SWD.P$1
SWDIO  (via drill 0.3 pad 0.6)
  Top 0.152: v24.04,12.28 23.78,12.01 23.72,11.95 U1.25
  Bottom 0.152: v24.04,12.28 23.63,12.28 23,12.91 23,15.12 24.34,16.45 SWD.P$3
TX-DOWNLOAD  (via drill 0.35)
  Top 0.152: R6.2 29.61,7.46 31.02,8.87 v33.05,8.87 U2.11
  Bottom 0.152: v33.05,8.87 33.05,10.58 TX.P$1
TYPE_C_D+  (via drill 0.3)
  Top 0.152: v5.27,9.85 5.48,9.64 TYPE-C1.B6 7.92,9.64 8.16,9.88 8.16,10.52 | 8.16,10.52 8.16,10.64 | R10.1 14.42,10.81 8.33,10.81 8.16,10.64 | 8.16,10.64 | TYPE-C1.A6 8.05,10.64 | 8.05,10.64 8.16,10.64 | 8.16,10.64 | 8.05,10.64 8.16,10.52 | 8.16,10.64
  Bottom 0.152: P1.P$1 2.07,10.24 4.88,10.24 v5.27,9.85
TYPE_C_D-  (via drill 0.3)
  Top 0.152: 5.3,10.68 5.3,10.81 5.63,11.14 TYPE-C1.B7 14.15,11.14 R11.1 | TYPE-C1.A7 5.74,10.14 5.3,10.58 5.3,10.68 | v5.31,10.69 5.3,10.68
  Bottom 0.152: P2.P$1 1.23,11.67 2.35,10.55 5.17,10.55 v5.31,10.69
USB_D+
  Top 0.152: 14.94,10.87 15.63,11.55 U1.47
  Top 0.203: 14.94,10.87 R10.2
USB_D-
  Top 0.152: U1.46 15.46,11.95 R11.2
VBUS  (2 unrouted)
  Top 0.254: 1.39,19.39 PICO-W.40-3 | TYPE-C1.B4 6.78,8.09 6.78,7.98 | TYPE-C1.A9 6.87,7.98 7.16,7.98 | 6.71,12.79 6.73,12.81 7.02,12.81 7.05,12.84 6.83,12.84 TYPE-C1.A4 TYPE-C1.B9
  Top 0.61: 1.39,19.39 1.38,19.38 D1.A 2.65,16.74 3.4,15.99 3.4,12.77 | 3.4,11.94 3.4,10.38 5.8,7.98 6.78,7.98 7.16,7.98 | 3.4,11.94 3.4,12.36 | 3.4,12.36 3.42,12.38 3.79,12.38 | 3.79,12.38 5.38,12.38 5.79,12.79 6.71,12.79 | 3.4,12.77 3.4,12.36 | 3.79,12.38 3.4,12.77 | 3.79,12.38 3.79,12.33 3.4,11.94
  Top 0.813: PICO-W.40-2 1.39,19.39
VSYS  (3 unrouted)
  Top 0.152: U4.1 18.13,17.59 18.36,17.59 | C9.2 17.01,17.64 17.03,17.63
  Top 0.508: 18.04,17.6 U4.1 | PICO-W.39-1 3.93,17.34 4.44,16.83 5.09,16.83 | 5.07,16.85 7.06,16.85 7.85,17.64 C9.2 | 18.24,17.46 18.36,17.59 | U4.1 18.06,17.58 17.97,17.58 17.93,17.63 | 15.55,17.58 C8.2 18,17.62 18.01,17.63 U4.1 | 18.13,17.59 18.09,17.63 17.03,17.63 16.37,17.63 C9.2 | R14.2 C9.2
  Top 0.61: D1.C 5.09,16.83 5.07,16.85

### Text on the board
bPlace: 3V3 | VBUS | VSYS | GND | GP28 | GND | GP27 | GP26 | GP22 | GND | GP21 | GP20 | GP19 | GP18 | GND | GP17 | GP16 | 3V3_EN | RESET | ADC_VREF | DM | DIO | Pico W5 | GND | V1.0 | DP | CMB12201R | CLK | BOOT | NC | NC | GND | GP0 | GP1 | GND | GP2 | GP3 | GND | GP6 | GP7 | GP8 | GP9 | GND | GP10 | GP11 | GP12 | GP13 | GP14 | GP15
tNames: LED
